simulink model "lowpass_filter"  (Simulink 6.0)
settings: Solver=ode45  StartTime=0.0  StopTime=10ms  RelTol=1e-3
PreLoadFcn:
  | coef
undefined symbols (not defined in the file or in its folder): C, dsp_flow, lab4, labs, netlist, training, Ts
libraries: xbsIndex_r3 x6, simulink x1, commnoisgen2 x1

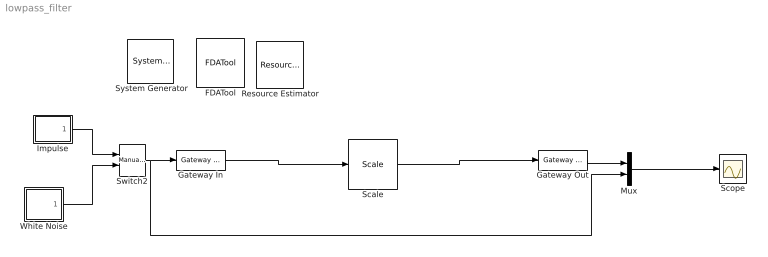
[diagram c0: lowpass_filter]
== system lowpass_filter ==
  " System Generator" : xbsIndex_r3/ System Generator  Tag=genX  xilinxfamily=Virtex2P  part=xc2vp4  speed=-7  package=fg456  synthesis_tool=XST  directory=./netlist  testbench=off  simulink_period=7.4074074074074073e-008  sysclk_period=10  incr_netlist=off  trim_vbits=Everywhere in SubSystem  dbl_ovrd=According to Block Masks  core_generation=According to Block Masks  run_coregen=off  deprecated_control=off  eval_field=0
  FDATool : xbsIndex_r3/FDATool
  Gateway In : xbsIndex_r3/Gateway In  arith_type="Signed  (2's comp)"  n_bits=8  bin_pt=6  quantization=Truncate  overflow=Wrap  period=1/1500000  timing_constraint=None  locs_specified=off  LOCs={}  needs_fixed_name=off  dbl_ovrd=off  show_param=off
  Gateway Out : xbsIndex_r3/Gateway Out  output_type=Double  nbits=8  bin_pt=6  arith_type=Boolean  quantization=Truncate  overflow=Wrap  hdl_port=on  timing_constraint=None  locs_specified=off  LOCs={}  needs_fixed_name=off  show_param=off
  Impulse : Subsystem
  Mux : Mux  Inputs=2
  Resource Estimator : xbsIndex_r3/Resource Estimator  Tag=resEstTag  xl_estimator_area=[304 502 0 439 0 0 0]  xl_use_estimator_area=off  simulink_period=7.4074074074074073e-008  mrp_directory=C:\training\dsp_flow\labs\lab4\netlist
  Scale : xbsIndex_r3/Scale  scale_factor=4  explicit_period=off  period=1  dbl_ovrd=off
  Scope : Scope
  Switch2 : simulink/Signal Routing/Manual Switch  sw=0  action=0
  White Noise : Subsystem
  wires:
  Gateway Out/1 -> Mux/1
  Mux/1 -> Scope/1
  White Noise/1(Out1) -> Switch2/2
  Impulse/1(Out1) -> Switch2/1
  Switch2/1 -> Gateway In/1, Mux/2
  Gateway In/1 -> Scale/1
  Scale/1 -> Gateway Out/1

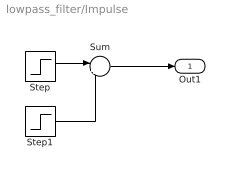
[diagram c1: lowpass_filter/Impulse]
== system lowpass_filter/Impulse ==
  Step : Step  Time=1*Ts  SampleTime=Ts
  Step1 : Step  Time=2*Ts  SampleTime=Ts
  Sum : Sum  Inputs=|+-
  Out1 : Outport
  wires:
  Step/1 -> Sum/1
  Sum/1 -> Out1/1
  Step1/1 -> Sum/2

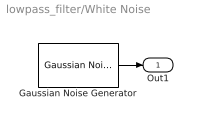
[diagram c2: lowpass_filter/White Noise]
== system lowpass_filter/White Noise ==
  Gaussian Noise Generator : commnoisgen2/Gaussian Noise Generator  m=[0]  d=[1]  s=[12345]  Ts=Ts  frameBased=off  sampPerFrame=1  orient=off
  Out1 : Outport
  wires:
  Gaussian Noise Generator/1 -> Out1/1
